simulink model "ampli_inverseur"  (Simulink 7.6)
settings: Solver=ode15s  StartTime=0.0  StopTime=1  MaxStep=0.00002  RelTol=1e-3
StopFcn:
  | load signaux.mat
  | subplot 211
  | plotyy(x(1,:),x(2,:),x(1,:),x(3,:))
  | title('montage ampli inverseur')
  | axis([0 1 -0.2 1.2])
  | grid
  | gtext('Band-Limited Op-Amp')
  | 
  | subplot 212
  | plotyy(x(1,:),x(2,:),x(1,:),x(4,:))
  | axis([0 1 -0.2 1.2])
  | grid
  | gtext('Finite Gain Op-Amp')
undefined symbols (not defined in the file or in its folder): sigbuilder_block
libraries: fl_lib x12, nesl_utility x4, elec_lib x2

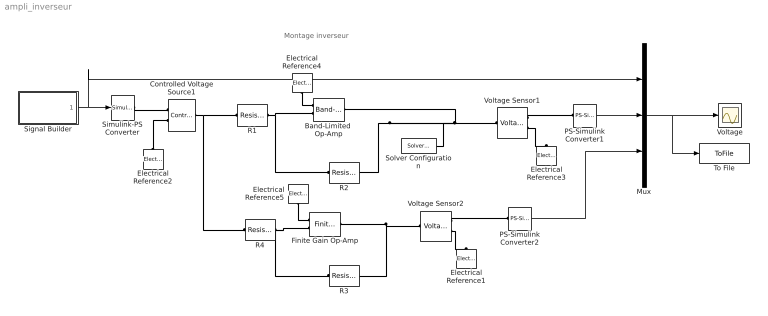
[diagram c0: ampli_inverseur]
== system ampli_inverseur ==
  note: Montage inverseur
  Band-Limited  Op-Amp : elec_lib/Integrated Circuits/Band-Limited Op-Amp  DialogController=NetworkEngine.DynNeDlgSource  SystemSampleTime=-1  A=1000  Rin=1e+06 Ohm  Rout=100 Ohm  Vmin=-15 V  Vmax=15 V  Vdotmax=1000 V/s  f=1e+05 Hz  V0=0 V  LocalVarNames=|power  LocalVarDescs=|Dissipated power (W)  LocalVarLogging=0
  Controlled Voltage Source1 : fl_lib/Electrical/Electrical Sources/Controlled Voltage Source  DialogController=NetworkEngine.DynNeDlgSource  SystemSampleTime=-1  i_Log=off  v_Log=off  LocalVarNames=|current|voltage|power  LocalVarDescs=|Current (A)|Voltage (V)|Power (W)  LocalVarLogging=[0 0 0]
  Electrical Reference{1..5} (5 alike) : fl_lib/Electrical/Electrical Elements/Electrical Reference  DialogController=NetworkEngine.DynNeDlgSource  SystemSampleTime=-1  i_Log=off  LocalVarNames=|i  LocalVarDescs=|i  LocalVarLogging=[]
  Finite Gain Op-Amp : elec_lib/Integrated Circuits/Finite Gain Op-Amp  DialogController=NetworkEngine.DynNeDlgSource  SystemSampleTime=-1  A=1000  Rin=1e+06 Ohm  Rout=100 Ohm  Vmin=-15 V  Vmax=15 V  LocalVarNames=|power  LocalVarDescs=|Dissipated power (W)  LocalVarLogging=0
  Mux : Mux  Inputs=3
  PS-Simulink Converter1 : nesl_utility/PS-Simulink Converter  DialogController=NetworkEngine.DynNeUtilDlgSource  SystemSampleTime=-1  PhysicalDomain=network_engine_domain  LeftPortType=input  RightPortType=output  SubClassName=ps_output  Unit=1  AffineConversion=off
  PS-Simulink Converter2 : nesl_utility/PS-Simulink Converter  DialogController=NetworkEngine.DynNeUtilDlgSource  SystemSampleTime=-1  PhysicalDomain=network_engine_domain  LeftPortType=input  RightPortType=output  SubClassName=ps_output  Unit=1  AffineConversion=off
  R1 : fl_lib/Electrical/Electrical Elements/Resistor  DialogController=NetworkEngine.DynNeDlgSource  SystemSampleTime=-1  R=1e3 Ohm  i_Log=off  v_Log=off  LocalVarNames=|current|voltage|power  LocalVarDescs=|Resistor current (A)|Voltage across resistor (V)|Power (W)  LocalVarLogging=[0 0 0]
  R2 : fl_lib/Electrical/Electrical Elements/Resistor  DialogController=NetworkEngine.DynNeDlgSource  SystemSampleTime=-1  R=0.5e3 Ohm  i_Log=off  v_Log=off  LocalVarNames=|current|voltage|power  LocalVarDescs=|Resistor current (A)|Voltage across resistor (V)|Power (W)  LocalVarLogging=[0 0 0]
  R3 : fl_lib/Electrical/Electrical Elements/Resistor  DialogController=NetworkEngine.DynNeDlgSource  SystemSampleTime=-1  R=0.5e3 Ohm  i_Log=off  v_Log=off  LocalVarNames=|current|voltage|power  LocalVarDescs=|Resistor current (A)|Voltage across resistor (V)|Power (W)  LocalVarLogging=[0 0 0]
  R4 : fl_lib/Electrical/Electrical Elements/Resistor  DialogController=NetworkEngine.DynNeDlgSource  SystemSampleTime=-1  R=1e3 Ohm  i_Log=off  v_Log=off  LocalVarNames=|current|voltage|power  LocalVarDescs=|Resistor current (A)|Voltage across resistor (V)|Power (W)  LocalVarLogging=[0 0 0]
  Signal Builder : Subsystem  Tag=STV Subsys  LoadFcn=sigbuilder_block('load');  StartFcn=sigbuilder_block('start');  StopFcn=sigbuilder_block('stop');  ClipboardFcn=sigbuilder_block('clipboard');
  Simulink-PS Converter : nesl_utility/Simulink-PS Converter  DialogController=NetworkEngine.DynNeUtilDlgSource  SystemSampleTime=-1  PhysicalDomain=network_engine_domain  LeftPortType=input  RightPortType=output  SubClassName=ps_input  Unit=1  AffineConversion=off  InputFilterTimeConstant=.001  UdotUserProvided=0
  Solver Configuration : nesl_utility/Solver Configuration  DialogController=NetworkEngine.DynNeUtilDlgSource  SystemSampleTime=-1  PhysicalDomain=network_engine_domain  LeftPortType=input  RightPortType=generic  SubClassName=solver  Accelerate=off  Profile=off  ResidualTolerance=1e-9  MaxNonlinIter=12  MaxModeIter=2  DoFixedCost=off  UseLocalSampling=off  DoDC=off  LinearAlgebra=Sparse  LocalSolverSampleTime=.001  LocalSolverChoice=NE_BACKWARD_EULER_ADVANCER  UseLocalSolver=off
  To File : ToFile  Filename=signaux  MatrixName=x
  Voltage : Scope
  Voltage Sensor1 : fl_lib/Electrical/Electrical Sensors/Voltage Sensor  DialogController=NetworkEngine.DynNeDlgSource  SystemSampleTime=-1  i1_Log=off  v1_Log=off  LocalVarNames=|i1|v1  LocalVarDescs=|i1|v1  LocalVarLogging=[]
  Voltage Sensor2 : fl_lib/Electrical/Electrical Sensors/Voltage Sensor  DialogController=NetworkEngine.DynNeDlgSource  SystemSampleTime=-1  i1_Log=off  v1_Log=off  LocalVarNames=|i1|v1  LocalVarDescs=|i1|v1  LocalVarLogging=[]
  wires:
  Mux/1 -> Voltage/1, To File/1
  Signal Builder/1(Signal 2) -> Simulink-PS Converter/1, Mux/1
  PS-Simulink Converter1/1 -> Mux/2
  PS-Simulink Converter2/1 -> Mux/3
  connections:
  Voltage Sensor1/RConn1 -- PS-Simulink Converter1/LConn1
  Simulink-PS Converter/RConn1 -- Controlled Voltage Source1/RConn1
  Electrical Reference2/LConn1 -- Controlled Voltage Source1/RConn2
  Voltage Sensor1/RConn2 -- Electrical Reference3/LConn1
  Electrical Reference4/LConn1 -- Band-Limited  Op-Amp/LConn1
  R1/RConn1 -- Band-Limited  Op-Amp/LConn2 -- R2/LConn1
  Controlled Voltage Source1/LConn1 -- R1/LConn1 -- R4/LConn1
  R2/RConn1 -- Band-Limited  Op-Amp/RConn1 -- Voltage Sensor1/LConn1 -- Solver Configuration/RConn1
  Voltage Sensor2/RConn2 -- Electrical Reference1/LConn1
  Voltage Sensor2/RConn1 -- PS-Simulink Converter2/LConn1
  R4/RConn1 -- Finite Gain Op-Amp/LConn2 -- R3/LConn1
  Electrical Reference5/LConn1 -- Finite Gain Op-Amp/LConn1
  Finite Gain Op-Amp/RConn1 -- Voltage Sensor2/LConn1 -- R3/RConn1

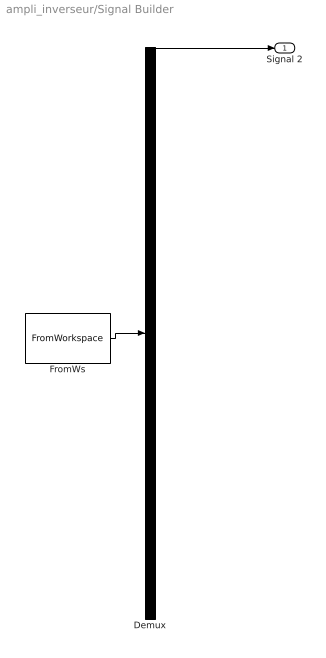
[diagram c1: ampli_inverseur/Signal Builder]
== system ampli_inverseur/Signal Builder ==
  Demux : Demux  Tag=STV Demux  Outputs=1
  FromWs : FromWorkspace  Tag=STV FromWs  VariableName=tuvar  SampleTime=0  SigBuilderData=DataTag0  VnvData=DataTag1
  Signal 2 : Outport  Tag=STV Outport
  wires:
  FromWs/1 -> Demux/1
  Demux/1 -> Signal 2/1
